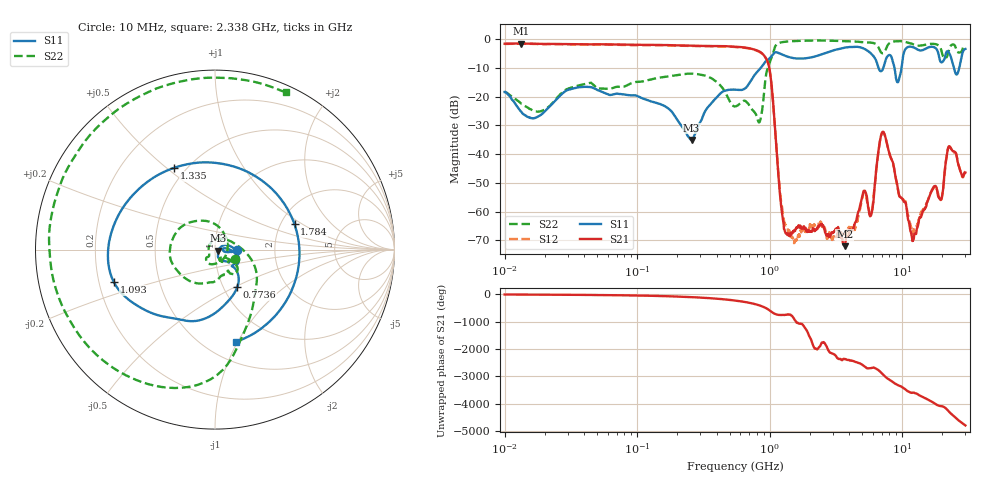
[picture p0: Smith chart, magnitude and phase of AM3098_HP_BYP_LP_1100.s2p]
!Agilent Technologies,E8364B,MY43040894,A.07.50.67
!Agilent E8364B: A.07.50.67
!Date: Wednesday, June 17, 2020 09:21:38
!Correction: S11(Full 2 Port(1,2))
!S21(Full 2 Port(1,2))
!S12(Full 2 Port(1,2))
!S22(Full 2 Port(1,2))
!S2P File: Measurements: S11, S21, S12, S22:Log Frequency Sweep
# Hz S  dB  R 50
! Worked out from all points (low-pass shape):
!   1601 points, 10 MHz to 30 GHz, reference 50 ohm
!   highest |S21| = -1.42 dB at 13.23 MHz (marker M1); lowest = -72.1 dB at 3.686 GHz (marker M2)
!   |S21| within 3 dB of the highest: start of sweep to 851.9 MHz
!   lowest |S11| = -35.1 dB at 257.3 MHz (marker M3), VSWR 1.04, Z = 51.7 - j0.621 ohm
!   |S11| at or under -10 dB: start of sweep to 854.3 MHz; 8.761 GHz to 9.887 GHz (1.127 GHz wide, 12.1 % of centre); 24.62 GHz to 26.93 GHz (2.311 GHz wide, 8.97 % of centre)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
!   |S22| runs from -28.9 to -0.4 dB; largest |S21 - S12| = 0.013
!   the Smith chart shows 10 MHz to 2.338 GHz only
!   S11 on the Smith chart (normalised r, x): 10 MHz: 1.28, -0.00; 773.6 MHz: 1.16, -0.51; 1.093 GHz: 0.26, -0.15; 1.335 GHz: 0.43, +0.53; 1.784 GHz: 2.37, +0.85; 2.338 GHz: 0.69, -0.99
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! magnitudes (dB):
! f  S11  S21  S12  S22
! 10 MHz  -18.3  -1.5  -1.6  -18.2
! 13.23 MHz  -25.1  -1.4  -1.5  -22.3
! 38.04 MHz  -16.6  -1.7  -1.7  -15.8
! 144.7 MHz  -22.3  -1.9  -2.0  -13.4
! 257.3 MHz  -35.1  -2.2  -2.3  -11.9
! 547.7 MHz  -17.5  -2.5  -2.6  -23.4
! 773.6 MHz  -12.3  -3.6  -3.6  -25.5
! 973.8 MHz  -7.1  -8.2  -8.3  -9.6
! 1.093 GHz  -4.6  -29.6  -29.8  -2.8
! 1.335 GHz  -5.9  -67.6  -64.9  -0.8
! 1.784 GHz  -6.7  -65.7  -66.0  -0.4
! 2.084 GHz  -6.2  -66.9  -64.6  -0.4
! 2.338 GHz  -5.6  -65.2  -64.9  -0.4
! 3.686 GHz  -2.9  -72.1  -68.0  -0.6
! 5.841 GHz  -5.0  -61.1  -60.7  -1.1
! 7.029 GHz  -10.9  -32.6  -32.7  -4.8
! 7.926 GHz  -5.5  -39.0  -39.1  -1.5
! 9.302 GHz  -14.9  -52.3  -52.5  -0.6
! 12.19 GHz  -2.8  -69.8  -67.1  -1.8
! 19.7 GHz  -7.9  -55.8  -55.8  -3.7
! 22.67 GHz  -4.8  -37.2  -37.5  -3.3
! 30 GHz  -3.3  -46.4  -46.1  -2.4
